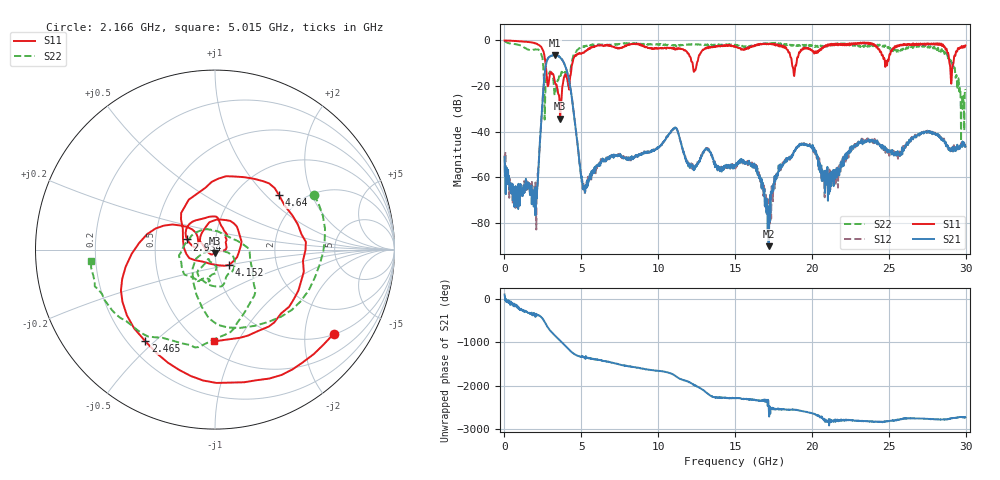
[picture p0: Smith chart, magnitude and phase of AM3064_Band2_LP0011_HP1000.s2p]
# Hz S DB R 50.0
!freq dBS11 angS11 dBS21 angS21 dBS12 angS12 dBS22 angS22
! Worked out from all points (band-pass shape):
!   1600 points, 10 MHz to 29.98 GHz, reference 50 ohm
!   highest |S21| = -6.39 dB at 3.29 GHz (marker M1); lowest = -90.2 dB at 17.18 GHz (marker M2)
!   |S21| within 3 dB of the highest: 2.744 GHz to 3.832 GHz (1.088 GHz wide, 33.1 % of centre)
!   lowest |S11| = -34.2 dB at 3.628 GHz (marker M3), VSWR 1.04, Z = 49.8 - j1.93 ohm
!   |S11| at or under -10 dB: 2.67 GHz to 4.419 GHz (1.748 GHz wide, 49.3 % of centre); 12.24 GHz to 12.52 GHz (279.5 MHz wide, 2.26 % of centre); 18.7 GHz to 19 GHz (298.4 MHz wide, 1.58 % of centre)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
!   |S22| runs from -44.2 to -0.2 dB; largest |S21 - S12| = 0.014
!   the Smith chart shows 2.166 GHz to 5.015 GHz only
!   S11 on the Smith chart (normalised r, x): 2.166 GHz: 1.02, -2.80; 2.465 GHz: 0.27, -0.47; 2.934 GHz: 0.73, +0.08; 4.152 GHz: 1.15, -0.20; 4.64 GHz: 1.55, +1.20; 5.015 GHz: 0.58, -0.81
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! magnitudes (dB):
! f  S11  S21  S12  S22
! 10 MHz  0.0  -51.1  -50.4  -0.2
! 778.5 MHz  -0.3  -65.9  -64.2  -1.7
! 2.166 GHz  -1.8  -62.3  -58.3  -4.0
! 2.465 GHz  -3.9  -27.5  -27.5  -7.6
! 2.934 GHz  -15.6  -7.2  -7.2  -13.9
! 3.29 GHz  -18.7  -6.4  -6.4  -23.6
! 3.628 GHz  -34.2  -7.5  -7.5  -15.5
! 4.152 GHz  -18.7  -15.9  -15.8  -19.8
! 4.64 GHz  -6.6  -39.0  -38.8  -5.1
! 5.015 GHz  -5.8  -59.6  -59.9  -3.2
! 10 GHz  -3.5  -47.0  -47.1  -1.8
! 11.11 GHz  -4.0  -38.4  -38.1  -2.2
! 15 GHz  -2.5  -55.4  -54.6  -1.8
! 16.3 GHz  -2.1  -55.3  -55.8  -2.0
! 17.18 GHz  -1.7  -90.2  -73.8  -1.5
! 17.97 GHz  -2.3  -55.5  -56.9  -1.3
! 19.99 GHz  -4.2  -46.8  -47.0  -2.0
! 21 GHz  -1.9  -55.5  -63.6  -2.7
! 23.1 GHz  -1.4  -44.6  -44.3  -2.2
! 25 GHz  -8.3  -48.5  -48.6  -2.8
! 28.56 GHz  -2.5  -44.0  -43.4  -4.6
! 29.98 GHz  -2.2  -46.4  -47.1  -21.7
